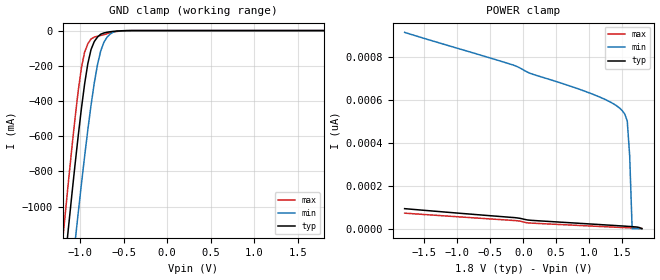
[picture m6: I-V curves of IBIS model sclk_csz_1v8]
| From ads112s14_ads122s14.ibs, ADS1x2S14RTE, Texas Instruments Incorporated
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|   Model sclk_csz_1v8
[Model] sclk_csz_1v8
Model_type Input
Polarity   Non-Inverting
Enable   Active-High
Vinl =  0.540V
Vinh =  1.260V
C_comp   1.000pF   0.500pF   2.000pF
[Model Spec]
Vinh   1.260V   1.155V   1.365V
Vinl   0.540V   0.495V   0.585V
[Temperature Range]   27.000   0.125k   -40.000
[Voltage Range]   1.800V   1.650V   1.950V
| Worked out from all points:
|   GND clamp passes 1 mA (typ) near -0.51 V on its own axis
[GND_clamp]
|Voltage   I(typ)   I(min)   I(max)
-1.8V     -4.321A    -4.211A    -4.387A
-1.208V   -1.482A    -1.911A    -1.228A
-1.171V   -1.298A    -1.732A    -1.039A
-1.134V   -1.117A    -1.554A    -853.4mA
-1.06V    -766mA     -1.207A    -501.9mA
-1.023V   -599.9mA   -1.038A    -344.6mA
-949mV    -303.3mA   -714.6mA   -122.5mA
-875mV    -107.5mA   -423.2mA   -47.74mA
-764mV    -20.72mA   -115.9mA   -27.81mA
-690mV    -9.399mA   -36.96mA   -17.74mA
-616mV    -4.409mA   -7.887mA   -8.375mA
1.8V      0A         0A         0A
[POWER_clamp]
|Voltage   I(typ)   I(min)   I(max)
-1.8V     93.02pA    912.5pA    72.11pA
-124mV    51.09pA    757.6pA    37.67pA
135mV     38.47pA    718.9pA    25.58pA
764mV     26.5pA     657.5pA    16.13pA
1.134V    19.53pA    615.2pA    10.66pA
1.356V    15.29pA    582.7pA    7.391pA
1.467V    13.13pA    559.2pA    5.762pA
1.541V    11.65pA    532.4pA    4.678pA
1.578V    10.89pA    500.5pA    4.136pA
1.615V    10.12pA    337.4pA    3.595pA
1.652V    9.318pA    0A         3.054pA
1.8V      0A         0A         888.4fA
